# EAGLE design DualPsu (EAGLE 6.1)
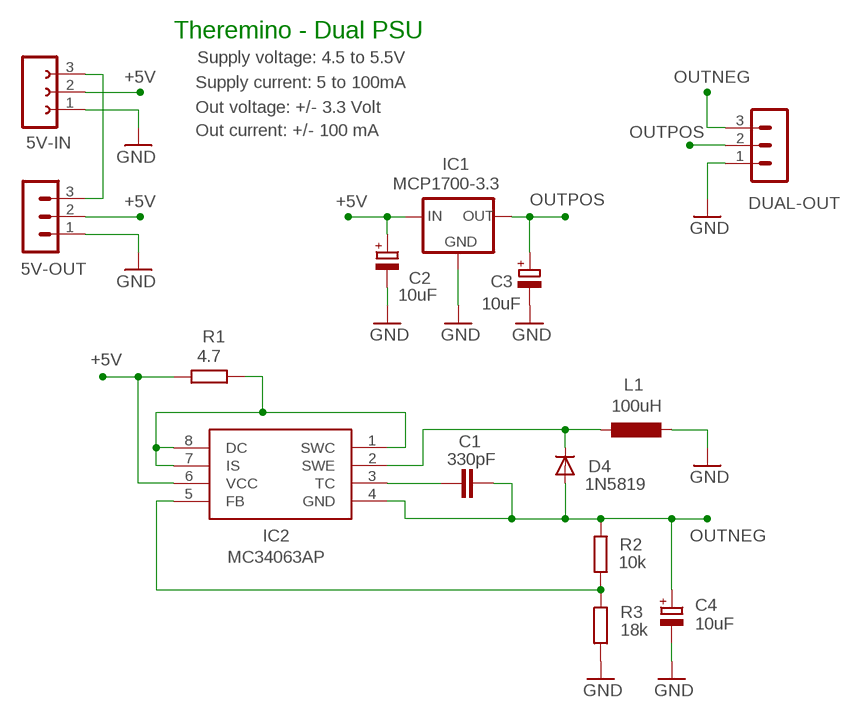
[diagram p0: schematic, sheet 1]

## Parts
5V-IN  FE03-1"  [FE03-1]
5V-OUT  MA03-1L3  [MA03-1_L3]
C1  330pF  C-EU025-024X044  [C025-024X044]
C2  10uF  CPOL-EUE2.5-5  [E2,5-5]
C3  10uF  CPOL-EUE2.5-5  [E2,5-5]
C4  10uF  CPOL-EUE2.5-5  [E2,5-5]
D4  1N5819  DIODE-DO34-7  [DO34-7]
DUAL-OUT  MA03-1L3  [MA03-1_L3]
IC1  MCP1700-3.3  MCP1700L1  [TO92L1]
IC2  MC34063AP  [DIL08]
L1  100uH  INDUCTORL_VERT_508  [L_VERT_508]
R1  4.7  R-EU_0204/7  [0204/7]
R2  10k  R-EU_0204/7  [0204/7]
R3  18k  R-EU_0204/7  [0204/7]

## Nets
+5V: 5V-IN.2 5V-OUT.2 C2.+ IC1.2(IN) IC2.6(VCC) R1.2
GND: 5V-IN.1 5V-OUT.1 C2.- C3.- C4.- DUAL-OUT.1 IC1.3(GND) L1.- R3.2
N$1: IC2.1(SWC) IC2.7(IS) IC2.8(DC) R1.1
N$2: C1.1 IC2.3(TC)
N$4: D4.C IC2.2(SWE) L1.+
N$5: 5V-IN.3 5V-OUT.3
N$6: IC2.5(FB) R2.1 R3.1
OUTNEG: C1.2 C4.+ D4.A DUAL-OUT.3 IC2.4(GND) R2.2
OUTPOS: C3.+ DUAL-OUT.2 IC1.1(OUT)

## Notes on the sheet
- Theremino - Dual PSU
- Supply voltage: 4.5 to 5.5V
- Supply current: 5 to 100mA
- Out voltage: +/- 3.3 Volt
- Out current: +/- 100 mA

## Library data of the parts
5V-IN = 02-con-lsta-F:FE03-1: FEMALE HEADER
5V-OUT DUAL-OUT = 03-con-lstb-M:MA03-1: PIN HEADER
C1 = 00-LIVIO:C-EU: CAPACITOR, European symbol
C2-C4 = 00-LIVIO:CPOL-EU: POLARIZED CAPACITOR, European symbol
D4 = 00-LIVIO:DIODE-: DIODE
IC1 = 00-LIVIO:MCP1700: Linear regulator Quescient courrent 1.8uA Input 2.3v to 6v Output 1.2v 1.8v 2.5v 3.0v 3.3v 5.0v
IC2 = 00-LIVIO:MC34063
L1 = 00-LIVIO:INDUCTOR
R1-R3 = 00-LIVIO:R-EU_: RESISTOR, European symbol

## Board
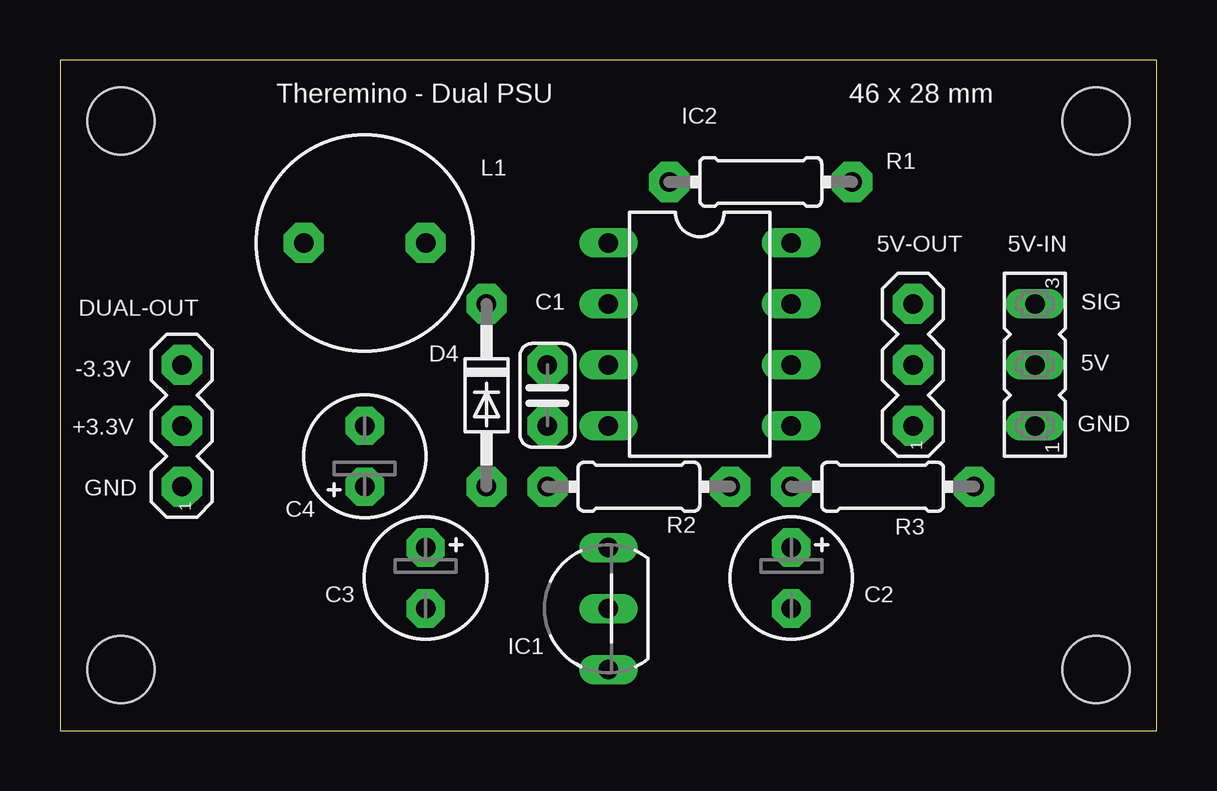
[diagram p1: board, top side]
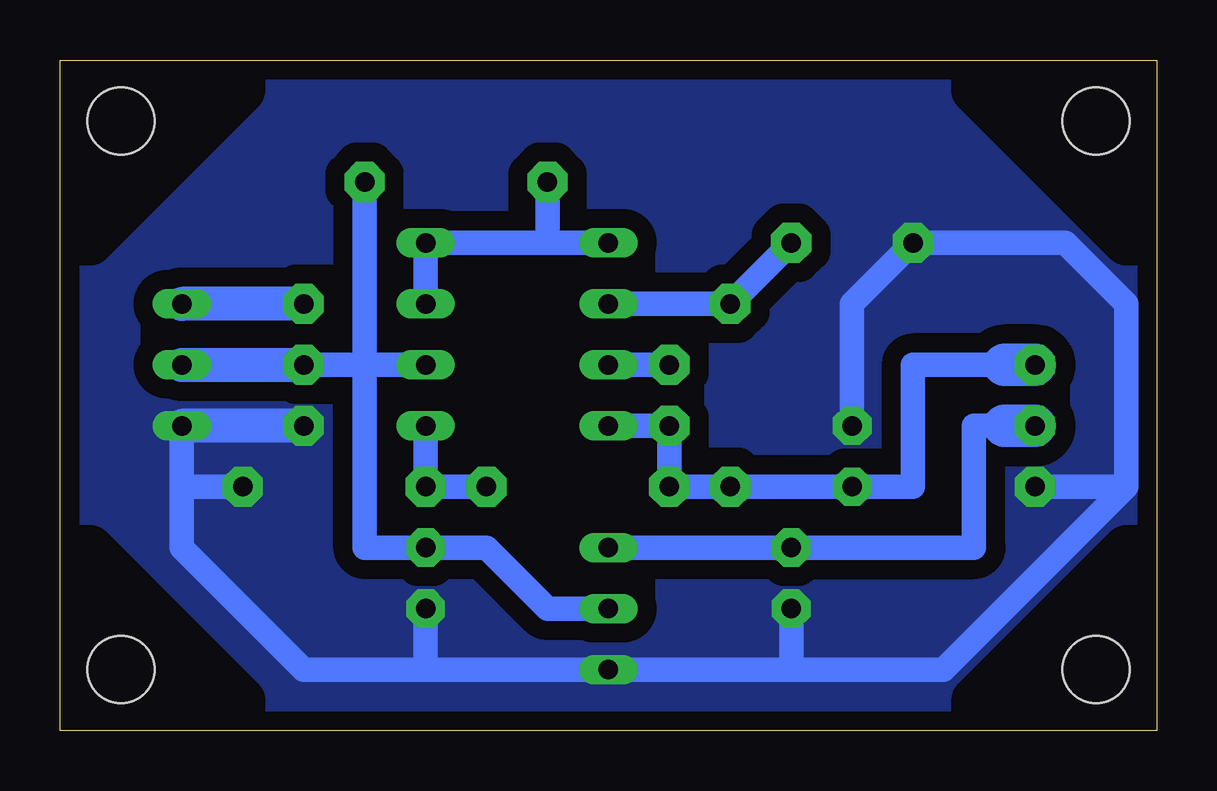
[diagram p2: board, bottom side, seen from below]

Size 45.72 x 27.94 mm. Coordinates in mm from the lower left corner, seen from the top.
Outline: 45.72,27.94 0,27.94 0,0 45.72,0 45.72,27.94
Copper layers (1*16): Top 0.035mm / dielectric 1.5mm / Bottom 0.035mm
Design rules: minimum track width 10mil, minimum drill 0.6mm, track to track 8mil, track to pad 8mil, pad to pad 8mil, via to via 8mil, smd to smd 8mil, copper to edge 31mil, drill to drill 8mil, minimum pad ring 5mil, minimum via ring 8mil, stop-mask expansion 4mil, vias tented up to drill 0mil, thermal gap 41mil
Holes 2.8 mm at 2.54,25.4 43.18,25.4 2.54,2.54 43.18,2.54
bRestrict: 4 lines

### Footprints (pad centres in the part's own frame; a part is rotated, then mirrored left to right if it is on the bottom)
FE03-1 = drill 0.813 long: 1 -2.54,0; 2 0,0; 3 2.54,0
MA03-1_L3 = drill 0.813 pad 1.676 octagon: 1 -2.54,0; 2 0,0; 3 2.54,0
C025-024X044 = drill 0.813 pad 1.676 octagon: 1 -1.27,0; 2 1.27,0
E2,5-5 = drill 0.813 pad 1.6 octagon: + -1.27,0; - 1.27,0
DO34-7 = drill 0.813 pad 1.676 octagon: A 3.81,0; C -3.81,0
TO92L1 = drill 0.813 long: 1 2.54,0; 2 0,0; 3 -2.54,0
DIL08 = drill 0.813 long: 1 -3.81,-3.81; 2 -1.27,-3.81; 3 1.27,-3.81; 4 3.81,-3.81; 5 3.81,3.81; 6 1.27,3.81; 7 -1.27,3.81; 8 -3.81,3.81
L_VERT_508 = drill 0.813 pad 1.676 octagon: + -2.54,0; - 2.54,0
0204/7 = drill 0.813 pad 1.676 octagon: 1 -3.81,0; 2 3.81,0

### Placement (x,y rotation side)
5V-IN  40.64,15.24 90 top
5V-OUT  35.56,15.24 90 top
C1  20.32,13.97 270 top
C2  30.48,6.35 270 top
C3  15.24,6.35 270 top
C4  12.7,11.43 90 top
D4  17.78,13.97 270 top
DUAL-OUT  5.08,12.7 90 top
IC1  22.86,5.08 90 top
IC2  26.67,16.51 270 top
L1  12.7,20.32 180 top
R1  29.21,22.86 0 top
R2  24.13,10.16 180 top
R3  34.29,10.16 0 top

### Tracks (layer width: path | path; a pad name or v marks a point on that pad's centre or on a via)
+5V
  Bottom 1.016: 5V-OUT.2 33.02,15.24 | 33.02,15.24 IC2.6 | R1.2 33.02,15.24 | IC1.2 25.4,5.08 27.94,7.62 C2.+ 33.02,7.62 33.02,15.24
  Bottom 1.422: 5V-IN.2 5V-OUT.2
GND
  Bottom 1.016: 1.27,10.16 1.27,17.78 3.81,20.32 L1.- 12.7,17.78 C4.- | DUAL-OUT.1 1.27,10.16 | C2.- 30.48,2.54 | 30.48,2.54 IC1.3 17.78,2.54 15.24,2.54 | 5V-IN.1 40.64,10.16 | 40.64,10.16 40.64,7.62 35.56,2.54 30.48,2.54 | 15.24,2.54 8.89,2.54 1.27,10.16 | C3.- 15.24,2.54 | R3.2 40.64,10.16
  Bottom 1.422: 5V-OUT.1 5V-IN.1
  pour Bottom (isolate 0.8, rank 6, no thermals): -1,-1 46.72,-1 46.72,28.94 -1,28.94
N$1
  Bottom 1.016: IC2.1 25.4,20.32 | 25.4,20.32 IC2.8 IC2.7 | R1.1 25.4,20.32
N$2
  Bottom 1.016: IC2.3 C1.1
N$4
  Bottom 1.016: IC2.2 D4.C L1.+
N$5
  Bottom 1.422: 5V-OUT.3 5V-IN.3
N$6
  Bottom 1.016: R2.1 R3.1 IC2.5
OUTNEG
  Bottom 1.016: IC2.4 C1.2 R2.2 D4.A C4.+ 10.16,10.16 10.16,15.24 6.35,15.24
  Bottom 1.778: DUAL-OUT.3 6.35,15.24
OUTPOS
  Bottom 1.016: IC1.1 C3.+ 7.62,7.62 7.62,12.7 6.35,12.7
  Bottom 1.778: 6.35,12.7 DUAL-OUT.2

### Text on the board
tNames: Theremino - Dual PSU | 46 x 28 mm | SIG | -3.3V | 5V | +3.3V | GND | GND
